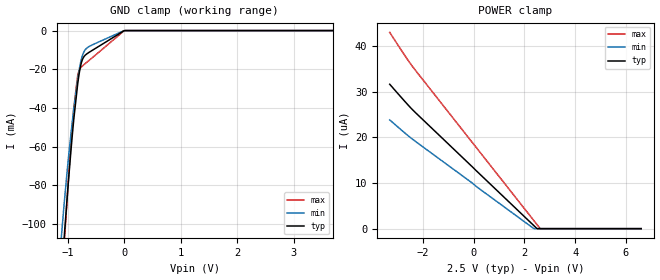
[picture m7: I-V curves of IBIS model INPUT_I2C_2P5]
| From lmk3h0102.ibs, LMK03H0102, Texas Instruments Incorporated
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[Model]   INPUT_I2C_2P5
Model_type   Input
Vinl = 0.75
Vinh = 1.75
|   typ   min   max
C_comp   0.7pF   0.5pF   0.9pF
[Voltage Range]   2.5   2.375   2.625
[Temperature Range]   45   125   -40
[Power Clamp Reference]   2.5   2.375   2.625
[GND Clamp Reference]   0   0   0
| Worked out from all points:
|   GND clamp passes 1 mA (typ) near -0.06 V on its own axis
[GND Clamp]
|   Voltage   I(typ)   I(min)   I(max)
-3.3V     -1.111A    -994.6mA   -1.235A
-1.181V   -155mA     -130.2mA   -166mA
-1.073V   -110.3mA   -92.21mA   -114.6mA
-1.063V   -106.3mA   -88.93mA   -110.1mA
-1.013V   -87.04mA   -73.2mA    -87.67mA
-943.8mV  -61.84mA   -53.24mA   -58.26mA
-894.3mV  -45.89mA   -40.53mA   -40.04mA
-815.1mV  -25.46mA   -23.28mA   -22mA
-755.7mV  -16.24mA   -14.37mA   -18.73mA
-676.5mV  -12.35mA   -9.42mA    -16.7mA
-3.3mV    -59.89uA   -42.63uA   -82.85uA
6.6V      0A         0A         0A
[POWER Clamp]
|   Voltage   I(typ)   I(min)   I(max)
-3.3V     31.6uA     23.8uA     42.95uA
-2.379V   25.9uA     19.48uA    35.31uA
2.373V    675.7nA    8.161nA    1.779uA
2.491V    44.94nA    0A         941.5nA
2.62V     0A         0A         33.83nA
6.6V      0A         0A         0A
